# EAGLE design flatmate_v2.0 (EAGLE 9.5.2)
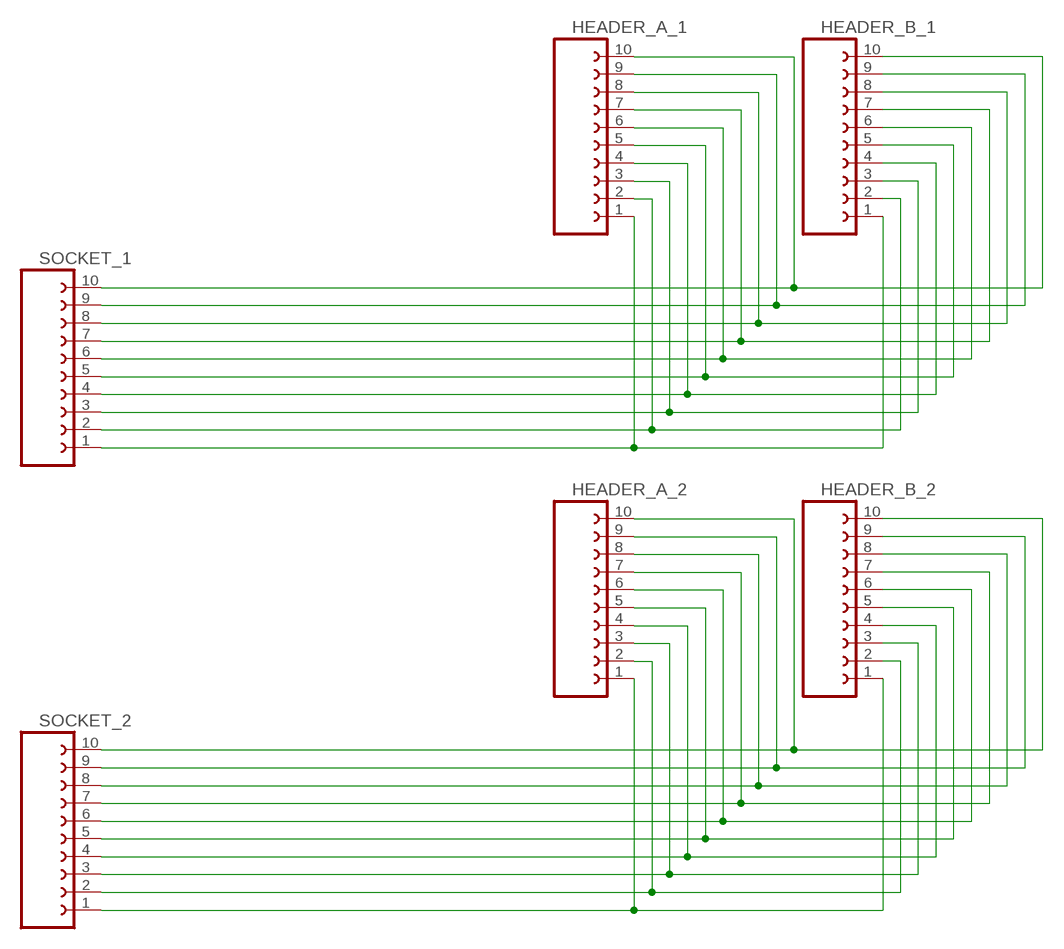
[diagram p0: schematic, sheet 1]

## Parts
HEADER_A_1  2MM_HEADER_1X10_SMD_B_DEV  [2MM_HEADER_1X10_SMD_B]
HEADER_A_2  2MM_HEADER_1X10_SMD_B_DEV  [2MM_HEADER_1X10_SMD_B]
HEADER_B_1  2MM_HEADER_1X10_SMD_B_DEV  [2MM_HEADER_1X10_SMD_B]
HEADER_B_2  2MM_HEADER_1X10_SMD_B_DEV  [2MM_HEADER_1X10_SMD_B]
SOCKET_1  2MM_SOCKET_1X10_SMD_A_DEV  [2MM_SOCKET_1X10_SMD_A]
SOCKET_2  2MM_SOCKET_1X10_SMD_A_DEV  [2MM_SOCKET_1X10_SMD_A]

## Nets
N$1: HEADER_A_1.1 HEADER_B_1.1 SOCKET_1.1
N$2: HEADER_A_1.2 HEADER_B_1.2 SOCKET_1.2
N$3: HEADER_A_1.3 HEADER_B_1.3 SOCKET_1.3
N$4: HEADER_A_1.5 HEADER_B_1.5 SOCKET_1.5
N$5: HEADER_A_1.4 HEADER_B_1.4 SOCKET_1.4
N$6: HEADER_A_2.1 HEADER_B_2.1 SOCKET_2.1
N$7: HEADER_A_1.6 HEADER_B_1.6 SOCKET_1.6
N$8: HEADER_A_2.2 HEADER_B_2.2 SOCKET_2.2
N$9: HEADER_A_2.3 HEADER_B_2.3 SOCKET_2.3
N$10: HEADER_A_1.7 HEADER_B_1.7 SOCKET_1.7
N$11: HEADER_A_2.4 HEADER_B_2.4 SOCKET_2.4
N$12: HEADER_A_2.5 HEADER_B_2.5 SOCKET_2.5
N$13: HEADER_A_1.8 HEADER_B_1.8 SOCKET_1.8
N$14: HEADER_A_2.6 HEADER_B_2.6 SOCKET_2.6
N$15: HEADER_A_2.7 HEADER_B_2.7 SOCKET_2.7
N$16: HEADER_A_1.9 HEADER_B_1.9 SOCKET_1.9
N$17: HEADER_A_2.8 HEADER_B_2.8 SOCKET_2.8
N$18: HEADER_A_2.9 HEADER_B_2.9 SOCKET_2.9
N$19: HEADER_A_1.10 HEADER_B_1.10 SOCKET_1.10
N$20: HEADER_A_2.10 HEADER_B_2.10 SOCKET_2.10

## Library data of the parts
HEADER_A_1 HEADER_A_2 HEADER_B_1 HEADER_B_2 = crazyflie:2MM_HEADER_1X10_SMD_B_DEV: 2mm header pin, alternating SMD pads (1x10)
SOCKET_1 SOCKET_2 = crazyflie:2MM_SOCKET_1X10_SMD_A_DEV: 2mm header pin socket, alternating SMD pads (1x10)

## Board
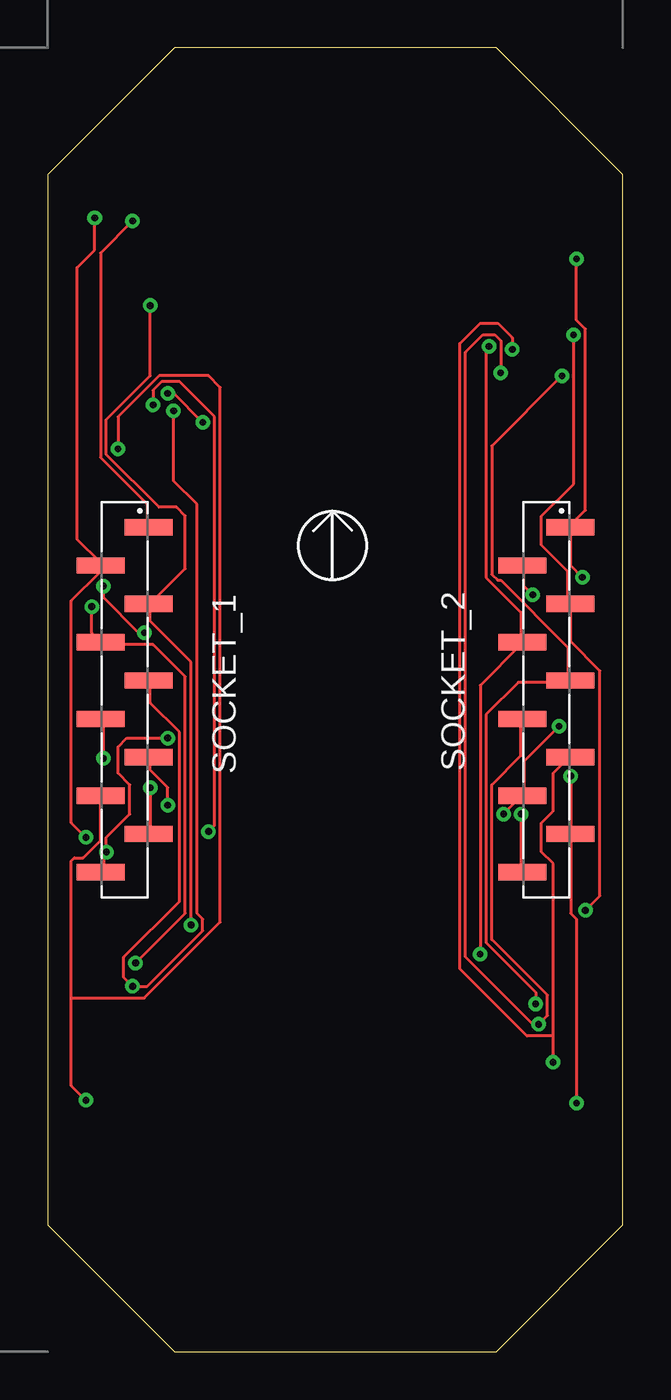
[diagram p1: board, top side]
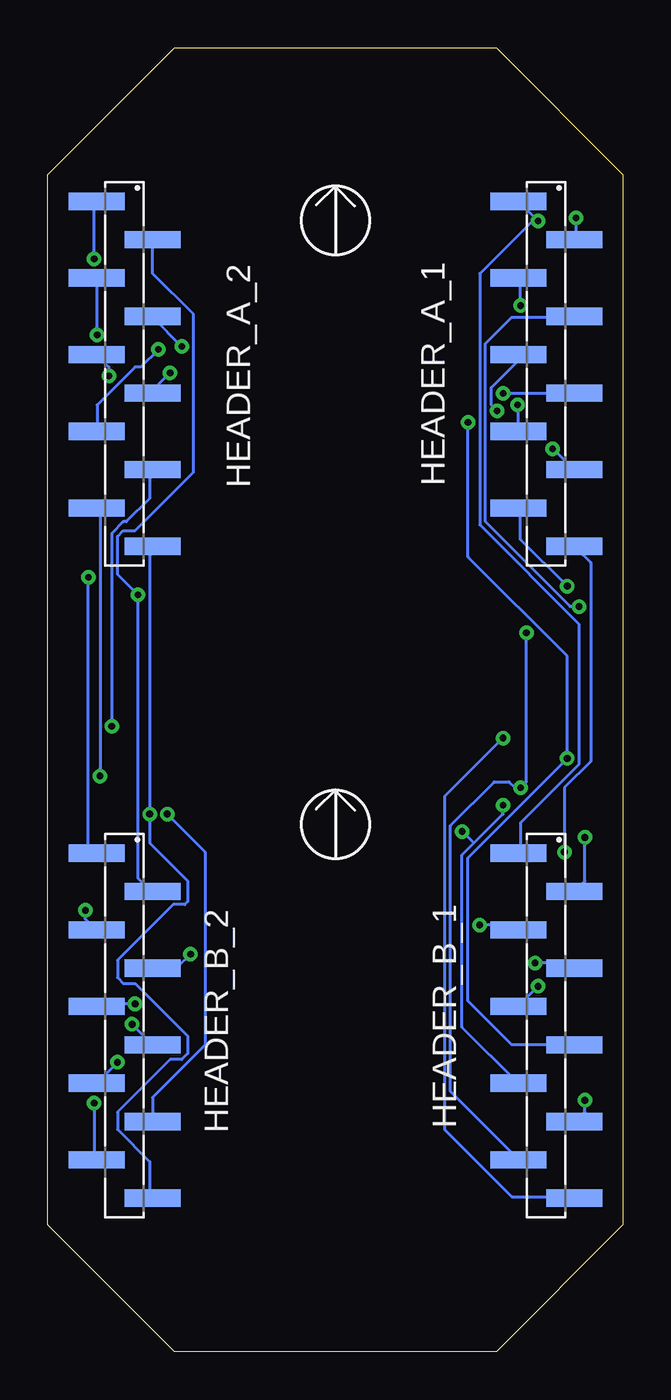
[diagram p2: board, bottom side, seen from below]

Size 30 x 68 mm. Coordinates in mm from the lower left corner, seen from the top.
Outline: 30,6.6 30,61.4 23.4,68 6.6,68 0,61.4 0,6.6 6.6,0 23.4,0 30,6.6
Copper layers (1*16): Top 0.035mm / dielectric 1.5mm / Bottom 0.035mm
Design rules "default": minimum track width 6mil, minimum drill 0.35mm, track to track 6mil, track to pad 6mil, pad to pad 6mil, via to via 6mil, smd to smd 6mil, copper to edge 40mil, drill to drill 6mil, minimum pad ring 10mil, minimum via ring 8mil, stop-mask expansion 4mil, vias tented up to drill 0mil, thermal gap 10mil

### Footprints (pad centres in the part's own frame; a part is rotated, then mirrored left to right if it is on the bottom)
2MM_HEADER_1X10_SMD_B = smd 0.9 x 2.92: 1 -1,-1.46; 2 1,1.46; 3 3,-1.46; 4 5,1.46; 5 7,-1.46; 6 9,1.46; 7 11,-1.46; 8 13,1.46; 9 15,-1.46; 10 17,1.46
2MM_SOCKET_1X10_SMD_A = smd 0.85 x 2.5: 1 -1,1.25; 2 1,-1.25; 3 3,1.25; 4 5,-1.25; 5 7,1.25; 6 9,-1.25; 7 11,1.25; 8 13,-1.25; 9 15,1.25; 10 17,-1.25

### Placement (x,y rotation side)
HEADER_A_1  4,59 270 bottom
HEADER_A_2  26,59 270 bottom
HEADER_B_1  4,25 270 bottom
HEADER_B_2  26,25 270 bottom
SOCKET_1  4,42 270 top
SOCKET_2  26,42 270 top

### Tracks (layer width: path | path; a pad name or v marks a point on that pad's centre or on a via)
N$1  (via drill 0.35)
  Top 0.152: v4.42,58.98 2.75,57.3 2.75,46.63 5.18,44.2 5.18,43.13 SOCKET_1.1
  Bottom 0.152: 4.57,59.13 5.34,59.89 HEADER_A_1.1 | 4.57,59.13 7.47,56.24 7.47,43.13 2.29,37.95 2.29,30.63 5.34,27.58 5.34,26.06 HEADER_B_1.1 | 4.57,59.13 v4.42,58.98
N$2  (via drill 0.35)
  Top 0.152: v1.98,26.82 1.22,27.58 1.22,39.17 2.75,40.69 SOCKET_1.2 2.75,41.15 1.53,42.37 1.53,56.54 2.44,57.45 v2.44,59.13
  Bottom 0.152: v1.98,26.82 1.98,24.54 2.44,24.08 HEADER_B_1.2 | v2.44,59.13 2.44,58.06 HEADER_A_1.2
N$3  (via drill 0.35)
  Top 0.152: v7.47,22.25 7.47,35.97 5.34,38.1 5.34,38.86 SOCKET_1.3 5.34,39.01 7.16,40.84 7.16,43.59 6.71,44.04 5.79,44.04 3.05,46.79 3.05,48.62 5.34,50.9 v5.34,54.56
  Bottom 0.152: v7.47,22.25 5.64,22.25 5.49,22.1 HEADER_B_1.3 | v5.34,54.56 5.34,55.93 HEADER_A_1.3
N$4  (via drill 0.35)
  Top 0.152: SOCKET_1.5 5.34,34.9 5.34,33.83 6.86,32.31 6.86,23.47 3.96,20.57 3.96,19.51 v4.42,19.05 5.18,19.05 8.08,21.95 8.08,22.55 7.77,22.86 7.77,44.2 6.55,45.41 v6.55,49.07
  Bottom 0.152: v4.42,19.05 5.34,18.14 HEADER_B_1.5 | v6.55,49.07 6.86,49.38 6.86,50.29 5.49,51.66 5.49,51.97 HEADER_A_1.5
N$5  (via drill 0.35)
  Top 0.152: v4.57,20.27 7.16,22.86 7.16,35.2 5.49,36.88 2.9,36.88 SOCKET_1.4 2.75,37.03 2.29,37.49 v2.29,38.86
  Bottom 0.152: v4.57,20.27 2.75,20.27 2.59,20.12 HEADER_B_1.4 | v2.29,38.86 2.75,38.86 7.16,43.28 7.16,52.58 5.79,53.95 2.59,53.95 HEADER_A_1.4
N$6  (via drill 0.35)
  Top 0.152: v27.89,40.39 27.28,41 27.28,42.98 SOCKET_2.1 27.28,43.13 28.04,43.89 28.04,53.34 27.59,53.8 v27.59,57
  Bottom 0.152: v27.89,40.39 27.89,26.36 27.59,26.06 HEADER_B_2.1 | v27.59,57 27.59,59.89 HEADER_A_2.1
N$7  (via drill 0.35)
  Top 0.152: v2.9,30.94 2.9,32.92 SOCKET_1.6 | v6.25,49.99 6.55,49.99 v8.08,48.46
  Bottom 0.152: HEADER_B_1.6 2.59,16 5.79,16 8.08,18.29 8.08,25.76 v2.9,30.94 2.9,36.27 8.08,41.45 v8.08,48.46 | v6.25,49.99 2.59,49.99 HEADER_A_1.6
N$8  (via drill 0.35)
  Top 0.152: v25.3,39.47 24.84,39.93 24.84,41 SOCKET_2.2
  Bottom 0.152: HEADER_B_2.2 24.69,24.08 25.3,24.69 v25.3,39.47 26.37,40.54 26.37,42.52 26.06,42.82 25.45,42.82 22.41,45.87 22.41,54.1 24.54,56.24 24.54,57.91 HEADER_A_2.2
N$9  (via drill 0.35)
  Top 0.152: v28.04,23.01 28.81,23.77 28.81,35.51 27.28,37.03 27.28,38.86 SOCKET_2.3 27.13,39.01 27.13,40.69 25.76,42.06 25.76,43.59 27.43,45.26 v27.43,53.03
  Bottom 0.152: v28.04,23.01 28.04,22.55 27.59,22.1 HEADER_B_2.3 | v27.43,53.03 27.43,55.93 HEADER_A_2.3
N$10  (via drill 0.35)
  Top 0.152: v6.25,28.5 6.25,29.41 5.34,30.33 5.34,30.94 SOCKET_1.7 | v5.49,49.38 5.49,50.14 5.95,50.6 6.86,50.6 8.69,48.77 8.69,27.43 v8.38,27.13
  Bottom 0.152: v6.25,28.5 6.25,28.04 7.77,26.52 | 7.77,26.52 8.38,25.91 8.38,16.92 5.49,14.02 HEADER_B_1.7 | v5.49,49.38 5.49,48.01 HEADER_A_1.7 | 7.77,26.52 v8.38,27.13
N$11  (via drill 0.35)
  Top 0.152: v23.01,52.43 22.86,52.27 22.86,40.39 24.69,38.56 24.69,37.03 SOCKET_2.4 24.69,36.88 22.56,34.75 v22.56,20.73
  Bottom 0.152: v23.01,52.43 24.54,53.95 HEADER_A_2.4 | v22.56,20.73 23.17,20.12 24.54,20.12 HEADER_B_2.4
N$12  (via drill 0.35)
  Top 0.152: v26.82,50.9 23.17,47.24 23.17,40.54 23.47,40.23 23.62,40.23 27.13,36.73 27.13,35.05 SOCKET_2.5 27.13,34.9 24.54,34.9 22.86,33.22 22.86,21.34 25.45,18.75 v25.45,18.14
  Bottom 0.152: v26.82,50.9 26.82,51.36 27.43,51.97 HEADER_A_2.5 | v25.45,18.14 27.43,18.14 HEADER_B_2.5
N$13  (via drill 0.35)
  Top 0.152: 1.22,18.44 1.22,13.87 v1.98,13.11 | 1.22,18.44 1.22,25.6 1.37,25.76 1.83,25.76 2.75,26.67 2.75,28.96 SOCKET_1.8 | v3.66,47.09 3.66,48.77 5.79,50.9 8.38,50.9 8.99,50.29 8.99,22.4 5.03,18.44 1.22,18.44
  Bottom 0.152: v1.98,13.11 1.98,12.5 2.44,12.04 HEADER_B_1.8 | v3.66,47.09 2.59,46.02 HEADER_A_1.8
N$14  (via drill 0.35)
  Top 0.152: SOCKET_2.6 24.69,32.92 24.69,31.09 23.17,29.57 23.17,21.49 26.06,18.59 26.06,17.53 v25.6,17.07 25.3,17.07 21.8,20.57 21.8,52.12 22.71,53.03 23.32,53.03 23.62,52.73 v23.62,51.05
  Bottom 0.152: v25.6,17.07 HEADER_B_2.6 | v23.62,51.05 24.54,50.14 HEADER_A_2.6
N$15  (via drill 0.35)
  Top 0.152: v26.37,15.09 26.37,16.46 | 26.37,16.46 26.37,25.45 25.76,26.06 25.76,27.58 26.37,28.19 26.37,30.18 27.13,30.94 SOCKET_2.7 | v24.23,52.27 24.23,52.88 23.47,53.65 22.56,53.65 21.49,52.58 21.49,19.96 25,16.46 26.37,16.46
  Bottom 0.152: v26.37,15.09 27.43,14.02 HEADER_B_2.7 | v24.23,52.27 25.15,51.36 25.45,51.36 27.43,49.38 27.43,48.01 HEADER_A_2.7
N$16  (via drill 0.35)
  Top 0.152: v5.34,29.41 5.34,27.13 SOCKET_1.9 | v2.9,39.93 2.9,39.32 4.73,37.49 v5.03,37.49
  Bottom 0.152: HEADER_B_1.9 5.49,10.06 8.99,13.56 8.99,27.43 6.71,29.72 5.95,29.72 5.64,29.41 v5.34,29.41 5.03,29.72 v5.03,37.49 | v2.9,39.93 5.34,42.37 5.34,43.89 HEADER_A_1.9
N$17  (via drill 0.35)
  Top 0.152: v26.67,32.61 24.84,30.79 24.84,29.11 SOCKET_2.8 24.69,28.96 v23.78,28.04
  Bottom 0.152: v26.67,32.61 26.67,42.67 26.06,43.28 25.91,43.28 24.69,44.5 24.69,45.87 HEADER_A_2.8 | v23.78,28.04 21.8,26.06 21.8,16 24.54,13.26 24.54,12.04 HEADER_B_2.8
N$18  (via drill 0.35)
  Top 0.152: v27.28,30.02 27.28,27.13 SOCKET_2.9 27.28,26.98 27.28,22.86 27.59,22.55 v27.59,12.95
  Bottom 0.152: v27.28,30.02 27.28,43.74 27.43,43.89 HEADER_A_2.9 | v27.59,12.95 27.59,10.06 HEADER_B_2.9
N$19  (via drill 0.35)
  Top 0.152: SOCKET_1.10 2.9,25.15 2.9,25.91 v3.05,26.06 3.05,26.82 4.27,28.04 4.27,29.57 3.66,30.18 3.66,31.55 4.12,32 v6.25,32
  Bottom 0.152: v3.05,26.06 3.05,29.41 1.68,30.79 1.68,41.15 2.44,41.91 HEADER_A_1.10 | v6.25,32 9.3,28.96 9.3,11.58 5.79,8.08 2.59,8.08 HEADER_B_1.10
N$20  (via drill 0.35)
  Top 0.152: v24.69,28.04 24.69,25.15 SOCKET_2.10
  Bottom 0.152: HEADER_A_2.10 24.69,41.91 v24.69,28.04 24.69,26.52 22.71,24.54 22.71,23.47 22.86,23.32 23.47,23.32 26.37,20.42 26.37,19.51 26.06,19.2 25.45,19.2 22.71,16.46 22.71,15.54 23.01,15.24 23.62,15.24 26.37,12.5 26.37,11.58 24.69,9.91 24.69,8.08 HEADER_B_2.10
